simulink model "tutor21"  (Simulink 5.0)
settings: Solver=ode45  SolverMode=SingleTasking  StartTime=0.0  StopTime=10  RelTol=1e-3  AbsTol=1e-3
libraries: simulink x1

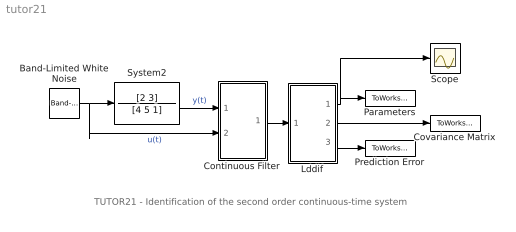
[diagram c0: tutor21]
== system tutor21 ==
  note: TUTOR21 - Identification of the second order continuous-time system
  Band-Limited White Noise : simulink/Sources/Band-Limited White Noise  Cov=[0.1]  Ts=0.1  seed=[23341]
  Continuous Filter : Subsystem  mask(C-Filter){par=[1,1], cit=[1], men=[2], tc=[1]}
      mask prompts: par "No. of inputs and outputs -  [in,out]:"; cit "Numerator degree -  [dn]:"; men "Denominator degree -  [dd]:"; tc "Time constant of the filter - [Tc]:"
      mask help: C-filter: Continuous filters Authors: Lubos Cirka and Miroslav Fikar 1998 - 2006
      mask init:
      | % State-space realisation of continuous-time MIMO filters
      | %
      | % Input:
      | %    y1(t), ..., yn(t), u1(t), ..., um(t)
      | % Output:
      | %    y(t), y'(t), y''(t) ..., u(t), u'(t), ...
      | 
      | % Calculation of the denominator with multiple time constant tc
      | 
      | in=par(1); out=par(2);
      | den=1;
      | for i=1:men,
      |    den=conv([tc 1],den);
      | end;
      | a=fliplr(den(2:men+1)/den(1));
      | 
      | % State-space realisation of the output filter
      | 
      | A0=zeros(out*(men-1),out);
      | A1=eye(out*(men-1));
      | for i=1:men
      |    A2(1:out,out*(i-1)+1:i*out)=-a(i)*eye(out);
      | end
      | Ay=[A0 A1;A2];
      | B0=zeros(out*(men-1),out);
      | B1=eye(out,out);
      | By=[B0;B1];
      | 
      | C0=-eye(out*(men-1)+out);C0(1:out,1:out)=eye(out);
      | for i=1:men
      |    C1(1:out,out*(i-1)+1:i*out)=a(i)*eye(out);
      | end
      | Cy=[C0;C1]/den(1);
      | Dy=-[zeros(out,out);By]/den(1);
      | 
      | % State-space realisation of the input filter
      | 
      | a0=zeros(in*(men-1),in);
      | a1=eye(in*(men-1));
      | for i=1:men
      |    a2(1:in,in*(i-1)+1:i*in)=-a(i)*eye(in);
      | end
      | Au=[a0 a1;a2];
      | b0=zeros(in*(men-1),in);
      | b1=eye(in,in);
      | Bu=[b0;b1];
      | if cit==men
      |    c0=eye(in*(cit-1)+in);
      |    for i=1:cit
      |       c1(1:in,in*(i-1)+1:i*in)=-a(i)*eye(in);
      |    end
      |    Cu=[c0;c1]/den(1);
      |    Du=[zeros(in*(cit-1)+in,in);eye(in)]/den(1);
      | else
      |    c0=eye(in*(cit+1));
      |    c1=zeros(in*(cit+1),(men-cit-1)*in);
      |    Cu=[c0 c1]/den(1);
      |    Du=zeros(in*(cit+1),in);
      | end
  Covariance Matrix : ToWorkspace  VariableName=CovMatrix  SaveFormat=Array
  Lddif : Subsystem  mask(LDDIF){par=[4,1], L=[0.985], d=[0.01], poc=[0 0 0 0], kov=[10e6], ts=[1]}
      mask prompts: par "No. of estimated parameters and outputs - [n,m]:"; L "Exponential forgetting - [L]:"; d "Bittanti's correction - [d]:"; poc "Initial parameter estimates - [theta(1) ... theta(n)]:"; kov "Covariance matrix (see help, standard - [10e6]):"; ts "Sampling period - [ts]:"
      mask help: LDDIF: + Bittanti's corrections Authors: Lubos Cirka and Miroslav Fikar 1998 - 2006
      mask init:
      | n=par(1); m=par(2);
  Parameters : ToWorkspace  VariableName=BA  SaveFormat=Array
  Prediction Error : ToWorkspace  VariableName=PredError  SaveFormat=Array
  Scope : Scope
  System2 : TransferFcn  Numerator=[2 3]  Denominator=[4 5 1]
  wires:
  Lddif/1(theta) -> Scope/1, Parameters/1
  Band-Limited White Noise/1 -> System2/1, Continuous Filter/2(u)  "u(t)"
  System2/1 -> Continuous Filter/1(y)  "y(t)"
  Continuous Filter/1("y, z") -> Lddif/1("y, z")
  Lddif/2(covariance matrix) -> Covariance Matrix/1
  Lddif/3(prediction error) -> Prediction Error/1

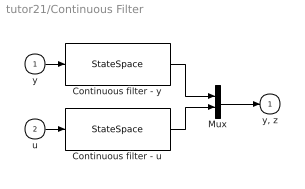
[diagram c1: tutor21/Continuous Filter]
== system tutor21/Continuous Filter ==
  y : Inport
  u : Inport  Port=2
  Continuous filter - u : StateSpace  A=Au  B=Bu  C=Cu  D=Du
  Continuous filter - y : StateSpace  A=Ay  B=By  C=Cy  D=Dy
  Mux : Mux  Inputs=2
  "y, z" : Outport  InitialOutput=0
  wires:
  y/1 -> Continuous filter - y/1
  u/1 -> Continuous filter - u/1
  Continuous filter - y/1 -> Mux/1
  Continuous filter - u/1 -> Mux/2
  Mux/1 -> "y, z"/1

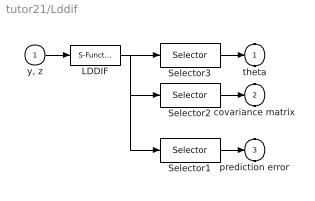
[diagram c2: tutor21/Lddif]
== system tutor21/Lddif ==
  "y, z" : Inport
  LDDIF : S-Function  FunctionName=lddif_s  Parameters=m, n, L, d, poc, kov, ts
  Selector1 : Selector  Elements=[n*m+n*n+1:1:n*m+n*n+m]  InputPortWidth=n*m+n*n+m
  Selector2 : Selector  Elements=[n*m+1:1:n*m+n*n]  InputPortWidth=n*m+n*n+m
  Selector3 : Selector  Elements=[1:1:n*m]  InputPortWidth=n*m+n*n+m
  theta : Outport  InitialOutput=0
  covariance matrix : Outport  Port=2  InitialOutput=0
  prediction error : Outport  Port=3  InitialOutput=0
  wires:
  Selector1/1 -> prediction error/1
  Selector3/1 -> theta/1
  Selector2/1 -> covariance matrix/1
  LDDIF/1 -> Selector1/1, Selector2/1, Selector3/1
  "y, z"/1 -> LDDIF/1
